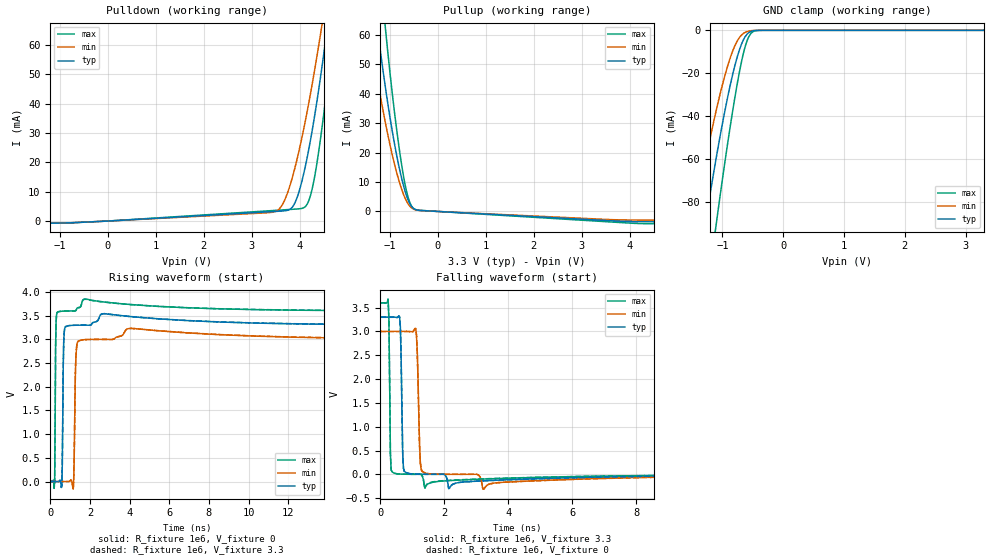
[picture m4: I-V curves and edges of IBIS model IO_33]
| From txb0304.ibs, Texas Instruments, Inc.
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[Model]   IO_33
Model_type  3-state
Enable   Active-High
Vref =   0
Rref =   1e6
Cref =   100p
Vmeas =   1.65
| variable   typ   min   max
C_comp   3.56pF   3.29pF   3.85pF
| C_pullup   3.85pF   3.56pF   4.00pF
| C_pulldown   3.84pF   3.56pF   3.99pF
| C_tri-state   3.56pF   3.29pF   3.85pF
[Temperature Range]   40   100   -40
| Ambient temperature   25   85   -40
[Voltage range]   3.3   3   3.6
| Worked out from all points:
|   slope of the pulldown table from 0 to 0.495 V, typ, clamps not added: 1.07 kohm
|   slope of the pullup table from 0 to 0.495 V, typ, clamps not added: 1.14 kohm
|   GND clamp passes 1 mA (typ) near -0.56 V on its own axis
|   rising waveform, R_fixture 1e6, V_fixture 0: 20-80 % time 50.1ps typ, 65.4ps min, 34.8ps max; typ from 0 V to 3.3 V
|   falling waveform, R_fixture 1e6, V_fixture 3.3: 20-80 % time 50.4ps typ, 65.2ps min, 36.2ps max; typ from 3.3 V to 0.004 V
|   rising waveform, R_fixture 1e6, V_fixture 3.3: 20-80 % time 50.2ps typ, 65.5ps min, 34.9ps max; typ from 0.004 V to 3.3 V
|   falling waveform, R_fixture 1e6, V_fixture 0: 20-80 % time 50.4ps typ, 65.2ps min, 36.2ps max; typ from 3.3 V to 0 V
[GND Clamp]
| IO_33
|   Voltage   I(typ)   I(min)   I(max)
-3.3V     -511mA     -429.4mA   -605.2mA
-1.49V    -128.8mA   -92.59mA   -176mA
-1.305V   -94.44mA   -64.67mA   -134.3mA
-1.27V    -88.18mA   -59.68mA   -126.6mA
-1.105V   -60.01mA   -37.73mA   -91.07mA
-955mV    -36.96mA   -20.66mA   -60.66mA
-835mV    -21.06mA   -9.955mA   -38.29mA
-710mV    -8.29mA    -2.997mA   -17.96mA
-620mV    -2.726mA   -874.7uA   -7.07mA
-530mV    -508.5uA   -191.3uA   -1.442mA
-410mV    -26.79uA   -12.71uA   -53.57uA
3.3V      1.562nA    31.41nA    89.95pA
[Pulldown]
| IO_33
|   Voltage   I(typ)   I(min)   I(max)
-3.3V     -1.028mA   -1.023mA   -1.025mA
-815mV    -630.7uA   -615.7uA   -648.4uA
3.485V    3.267mA    3.205mA    3.624mA
3.655V    3.441mA    6.112mA    3.801mA
3.85V     4.84mA     15.1mA     4.004mA
4.065V    14.93mA    29.97mA    4.414mA
4.155V    21.66mA    37.35mA    5.783mA
4.25V     29.98mA    45.77mA    10.36mA
4.445V    50.39mA    64.91mA    29.52mA
4.555V    63.61mA    76.67mA    43.91mA
4.7V      82.64mA    93.11mA    66.02mA
6.6V      425.9mA    369mA      508.5mA
[Pullup]
| IO_33
|   Voltage   I(typ)   I(min)   I(max)
-3.3V     431.1mA    323.4mA    596mA
-1.45V    88.21mA    64.14mA    129.7mA
-1.415V   83.2mA     60.43mA    122.5mA
-1.275V   64.18mA    46.37mA    94.71mA
-1.245V   60.32mA    43.53mA    89.06mA
-1.09V    41.78mA    29.87mA    61.69mA
-910mV    23.55mA    16.47mA    34.53mA
-745mV    10.61mA    7.093mA    14.83mA
-615mV    3.694mA    2.454mA    4.531mA
-495mV    888.1uA    700.1uA    897.5uA
4.12V     -3.46mA    -2.92mA    -4.061mA
6.6V      -3.647mA   -2.986mA   -4.405mA
[Ramp]
| IO_33
| variable   typ   min   max
dV/dt_r   2.21/5.68E-11   2.04/8.34E-11   2.40/3.94E-11
dV/dt_f   2.17/5.60E-11   2.02/7.76E-11   2.38/3.71E-11
R_load = 1e6
[Rising Waveform]
| IO_33
R_fixture =   1e6
C_fixture =   0
L_fixture =   0
V_fixture =   0
V_fixture_min = 0
V_fixture_max = 0
|   Time   V(typ)   V(min)   V(max)
0s        734nV      3.093uV    102.6nV
221ps     -84.65uV   2.95uV     24.78mV
269ps     -2.124uV   2.732uV    2.863V
317ps     181.8uV    2.51uV     3.519V
581ps     -108.4mV   -11.38uV   3.594V
725ps     3.226V     -41.17uV   3.597V
1.157ns   3.296V     -160.5mV   3.599V
1.325ns   3.298V     2.833V     3.636V
1.733ns   3.299V     2.993V     3.85V
117.8ns   3.296V     2.996V     3.596V
[Falling Waveform]
| IO_33
R_fixture =   1e6
C_fixture =   0
L_fixture =   0
V_fixture =   3.3
V_fixture_min = 3
V_fixture_max = 3.6
|   Time   V(typ)   V(min)   V(max)
0s        3.3V       3V         3.6V
245ps     3.3V       3V         3.678V
317ps     3.3V       3V         420.4mV
341ps     3.3V       3V         88.84mV
605ps     3.304V     3V         6.296mV
725ps     130mV      3V         3.184mV
1.109ns   4.256mV    3.062V     629.7uV
1.253ns   2.107mV    246mV      1.545mV
1.397ns   1.161mV    30.86mV    -287.5mV
117.8ns   3.511mV    3.525mV    3.462mV
[Rising Waveform]
| IO_33
R_fixture =   1e6
C_fixture =   0
L_fixture =   0
V_fixture =   3.3
V_fixture_min = 3
V_fixture_max = 3.6
|   Time   V(typ)   V(min)   V(max)
0s        3.501mV    3.512mV    3.456mV
221ps     3.413mV    3.512mV    28.15mV
269ps     3.495mV    3.511mV    2.864V
317ps     3.679mV    3.511mV    3.519V
581ps     -105mV     3.494mV    3.594V
725ps     3.226V     3.463mV    3.597V
1.157ns   3.296V     -157mV     3.599V
1.325ns   3.298V     2.833V     3.635V
1.757ns   3.299V     2.994V     3.846V
117.8ns   3.3V       3V         3.6V
[Falling Waveform]
| IO_33
R_fixture =   1e6
C_fixture =   0
L_fixture =   0
V_fixture =   0
V_fixture_min = 0
V_fixture_max = 0
|   Time   V(typ)   V(min)   V(max)
0s        3.296V     2.996V     3.596V
245ps     3.296V     2.996V     3.675V
317ps     3.296V     2.996V     418.8mV
341ps     3.296V     2.996V     88.65mV
605ps     3.301V     2.996V     6.279mV
725ps     129.6mV    2.996V     3.17mV
1.109ns   4.244mV    3.058V     627.2uV
1.253ns   2.098mV    245mV      1.64mV
1.397ns   1.153mV    30.81mV    -285.4mV
117.8ns   10.62uV    17.34uV    6.199uV
